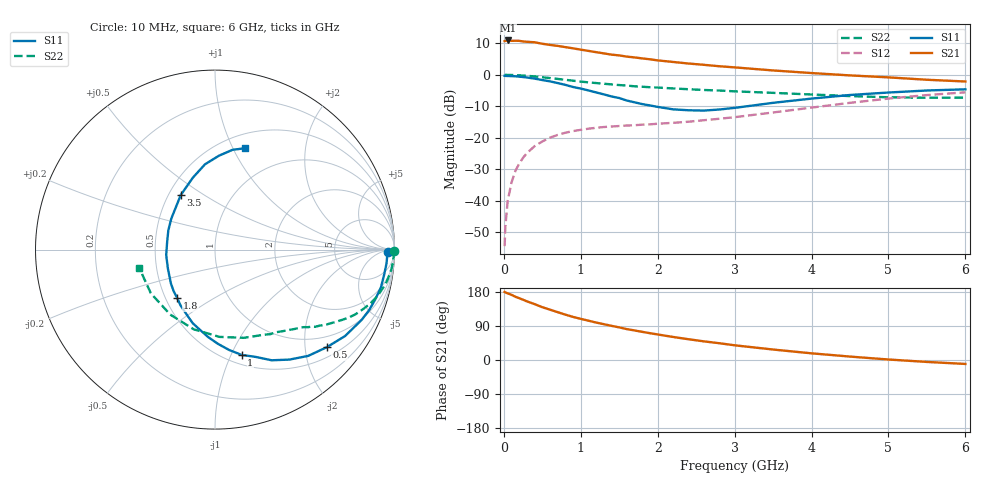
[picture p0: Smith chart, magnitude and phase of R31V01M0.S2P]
! SIEMENS Small Signal Semiconductors
! BFR181
! Si NPN RF Bipolar Junction Transistor in SOT23
! VCE = 1 V  IC = 1 mA
! Common Emitter S-Parameters:  May  1996
# GHz  S  MA  R  50
!  f  S11  S21  S12  S22
! GHz  MAG  ANG  MAG  ANG  MAG  ANG  MAG  ANG
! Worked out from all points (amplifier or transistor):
!   36 points, 10 MHz to 6 GHz, reference 50 ohm
!   highest |S21| = 10.9 dB at 50 MHz (marker M1)
!   |S21| within 3 dB of that: start of sweep to 1.019 GHz
!   unconditionally stable (mu >= 1): 1.918 GHz to 3.913 GHz
!   at 250 MHz: K = 0.16, MSG = 18.5 dB, |S12| = -26.3 dB
!   at 1.4 GHz: K = 0.79, MSG = 11.4 dB, |S12| = -16.4 dB
!   at 6 GHz: K = 0.92, MSG = 1.7 dB, |S12| = -5.6 dB
!   S11 on the Smith chart (normalised r, x): 10 MHz: 45, -19; 500 MHz: 0.72, -2.48; 1 GHz: 0.59, -1.10; 1.8 GHz: 0.57, -0.35; 3.5 GHz: 0.58, +0.40; 6 GHz: 0.64, +1.11
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0.01  0.963 -0.9  3.439 179.6  0.0019 93.8  0.9985 -0.4
0.02  0.9605 -1.6  3.453 178.3  0.0039 83.1  0.9985 -0.9
0.05  0.9588 -4.6  3.514 175.9  0.01 87.3  0.9963 -2.1
0.1  0.9528 -8.4  3.466 172.0  0.0195 84.7  0.9937 -4.2
0.15  0.9482 -12.8  3.476 166.9  0.0298 80.7  0.9891 -6.3
0.2  0.9351 -17.2  3.464 163.1  0.0389 78.5  0.9818 -8.3
0.3  0.9061 -25.6  3.349 154.7  0.0571 73.9  0.9651 -12.1
0.4  0.8701 -33.6  3.29 147.5  0.0736 68.8  0.9429 -15.8
0.5  0.8265 -41.2  3.115 139.4  0.0874 64.1  0.9156 -19.2
0.7  0.74 -55.9  2.88 126.2  0.1111 56.3  0.861 -24.8
0.9  0.6403 -69.1  2.634 113.7  0.1278 50.5  0.8059 -29.2
1  0.6052 -75.8  2.509 108.6  0.1337 48.1  0.7802 -31.2
1.1  0.5647 -82.0  2.399 103.7  0.1394 46.2  0.7595 -32.9
1.4  0.4533 -100.9  2.092 90.1  0.151 41.9  0.7051 -37.6
1.6  0.39 -114.7  1.945 81.5  0.1567 40.7  0.6751 -39.8
1.8  0.3427 -127.9  1.822 74.3  0.1618 41.0  0.6463 -42.2
2.2  0.283 -158.0  1.601 60.8  0.1728 42.0  0.6078 -47.5
3  0.2985 144.7  1.313 38.8  0.2124 46.3  0.5466 -60.3
3.5  0.359 122.1  1.173 27.6  0.2524 47.2  0.5172 -71.9
4.5  0.4784 96.7  0.979 9.0  0.3592 42.5  0.4597 -104.9
5.5  0.564 80.1  0.835 -5.1  0.4767 30.2  0.4325 -145.7
6  0.5887 73.6  0.783 -10.4  0.5273 22.6  0.4343 -166.5
